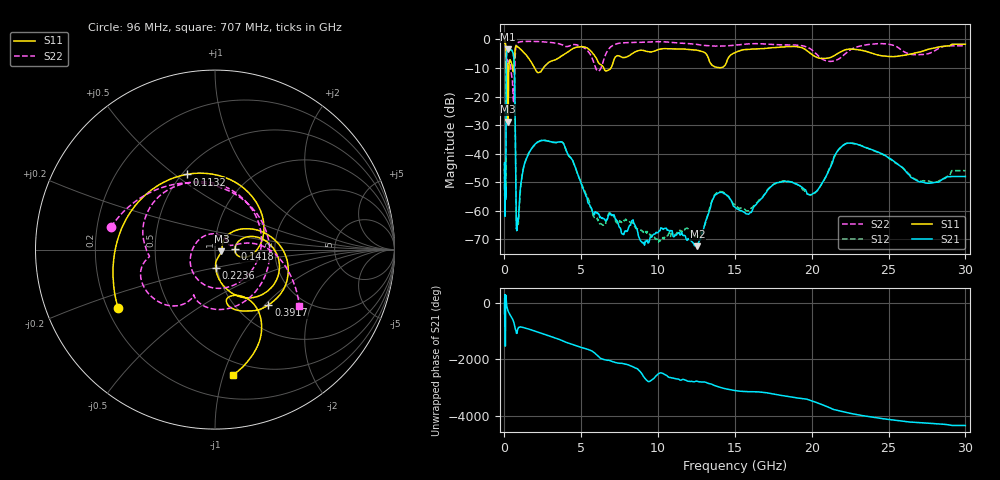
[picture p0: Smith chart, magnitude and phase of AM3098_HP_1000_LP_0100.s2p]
! Date/Time: Thu, Feb 28, 2019 8:39 AM
! Network Analyzer: Agilent Technologies E8364B Rev: A.07.50.67
! Sweep from 0.010 to 30.000 GHz, 1601 Points, Sweep Type: LOG
! Power Supply: 5.022 V, 0.002 A
# Hz S DB R 50
!freq MagS11 AngS11 MagS21 AngS21 MagS12 AngS12 MagS22 AngS22
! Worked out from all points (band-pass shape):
!   1601 points, 10 MHz to 30 GHz, reference 50 ohm
!   highest |S21| = -3.32 dB at 235.1 MHz (marker M1); lowest = -72.4 dB at 12.56 GHz (marker M2)
!   |S21| within 3 dB of the highest: 127.2 MHz to 605.3 MHz (478.1 MHz wide, 131 % of centre)
!   lowest |S11| = -28.7 dB at 237.5 MHz (marker M3), VSWR 1.08, Z = 53.7 - j0.951 ohm
!   |S11| at or under -10 dB: 198.6 MHz to 288.1 MHz (89.48 MHz wide, 36.8 % of centre); 1.958 GHz to 2.531 GHz (572.4 MHz wide, 25.5 % of centre); 6.467 GHz to 6.929 GHz (462.2 MHz wide, 6.9 % of centre)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
!   |S22| runs from -21.8 to -0.6 dB; largest |S21 - S12| = 0.013
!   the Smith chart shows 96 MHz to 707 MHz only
!   S11 on the Smith chart (normalised r, x): 96 MHz: 0.24, -0.26; 113.2 MHz: 0.53, +0.55; 141.8 MHz: 1.25, +0.01; 223.6 MHz: 0.99, -0.20; 391.7 MHz: 1.38, -1.05; 707 MHz: 0.39, -1.08
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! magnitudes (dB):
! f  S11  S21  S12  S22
! 10 MHz  -0.3  -43.9  -45.3  -0.6
! 38.04 MHz  -0.5  -58.7  -60.5  -0.8
! 82.62 MHz  -2.2  -53.3  -53.6  -2.5
! 96 MHz  -4.0  -41.7  -41.9  -4.5
! 113.2 MHz  -7.0  -15.7  -15.7  -10.3
! 141.8 MHz  -19.1  -4.4  -4.4  -10.8
! 144.7 MHz  -18.5  -4.3  -4.3  -10.4
! 183.1 MHz  -8.4  -3.9  -3.9  -7.0
! 223.6 MHz  -19.8  -3.4  -3.4  -8.5
! 235.1 MHz  -28.6  -3.3  -3.3  -8.7
! 237.5 MHz  -28.7  -3.3  -3.3  -8.7
! 391.7 MHz  -7.4  -3.6  -3.6  -9.3
! 550.5 MHz  -10.9  -4.6  -4.6  -18.5
! 646.1 MHz  -6.7  -10.4  -10.3  -15.5
! 707 MHz  -3.0  -34.0  -33.7  -5.0
! 805.2 MHz  -2.3  -66.8  -64.2  -1.5
! 2.084 GHz  -11.2  -36.2  -36.3  -0.7
! 3.779 GHz  -5.5  -36.1  -36.0  -1.9
! 7.926 GHz  -6.2  -67.1  -63.2  -1.1
! 12.56 GHz  -3.8  -72.4  -69.1  -1.8
! 22.56 GHz  -3.4  -36.3  -36.3  -3.5
! 30 GHz  -1.7  -48.0  -46.0  -2.2
